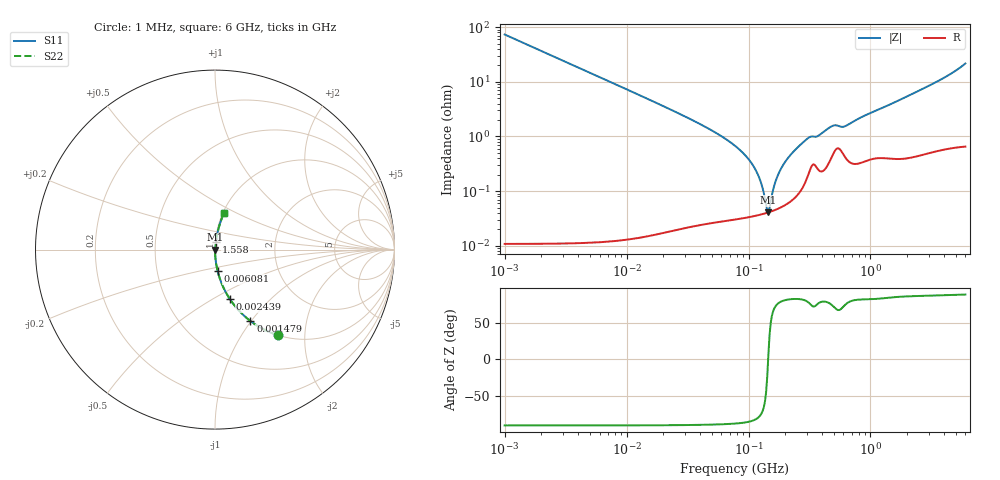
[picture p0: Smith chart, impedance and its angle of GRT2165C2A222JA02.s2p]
!Murata Part Number: GRT2165C2A222JA02
!These Parameters are Measured in Series Mode Connection
!Data Generated on Jun 19, 2026
!  o--ll--o
!Port1  Port2
!  o------o
!Operation Temp=25[degC], DC Bias Voltage=0[V]
!Freq. Start=1000[kHz] Stop=6[GHz] 401[Steps]
# Hz S RI R 50
!Freq.(Hz) S11(Real) S11(Imag) S21(Real) S21(Imag) S12(Real) S12(Imag) S22(Real) S22(Imag)
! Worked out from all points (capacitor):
!   401 points, 1 MHz to 6 GHz, reference 50 ohm
!   read as one part in series: C = 2.17 nF near 1.044 MHz
!   lowest |Z| = 41.2 mohm at 145.5 MHz (marker M1)
!   series resonance near 144.9 MHz, so ESL is about 560 pH
!   S11 on the Smith chart (normalised r, x): 1 MHz: 1.00, -1.47; 1.479 MHz: 1.00, -0.99; 2.439 MHz: 1.00, -0.60; 6.081 MHz: 1.00, -0.24; 1.558 GHz: 1.01, +0.08; 6 GHz: 1.01, +0.43
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1000000  0.35 -0.4769  0.65 0.4769  0.65 0.4769  0.35 -0.4769
1479166  0.1975 -0.398  0.8025 0.398  0.8025 0.398  0.1975 -0.398
2439274  0.083 -0.2758  0.917 0.2758  0.917 0.2758  0.083 -0.2758
4293785  0.0284 -0.1659  0.9716 0.1659  0.9716 0.1659  0.0284 -0.1659
6080879  0.0144 -0.1187  0.9856 0.1187  0.9856 0.1187  0.0144 -0.1187
1.843659e7  0.00169 -0.039  0.9983 0.039  0.9983 0.039  0.00169 -0.039
4.596069e7  0.000457 -0.0143  0.9995 0.0143  0.9995 0.0143  0.000457 -0.0143
7.745967e7  0.000348 -0.00674  0.9997 0.00674  0.9997 0.00674  0.000348 -0.00674
9.83954e7  0.000347 -0.00401  0.9997 0.00401  0.9997 0.00401  0.000347 -0.00401
1.145757e8  0.00036 -0.0024  0.9996 0.0024  0.9996 0.0024  0.00036 -0.0024
1.277378e8  0.000378 -0.00128  0.9996 0.00128  0.9996 0.00128  0.000378 -0.00128
1.39348e8  0.000397 -0.000394  0.9996 0.000394  0.9996 0.000394  0.000397 -0.000394
1.455431e8  0.000409 4.89e-05  0.9996 -4.89e-05  0.9996 -4.89e-05  0.000409 4.89e-05
1.694764e8  0.000466 0.00162  0.9995 -0.00162  0.9995 -0.00162  0.000466 0.00162
1.930997e8  0.000542 0.00301  0.9995 -0.00301  0.9995 -0.00301  0.000542 0.00301
2.506837e8  0.000874 0.00613  0.9991 -0.00613  0.9991 -0.00613  0.000874 0.00613
3.325952e8  0.00306 0.00951  0.9969 -0.00951  0.9969 -0.00951  0.00306 0.00951
4.919634e8  0.00487 0.0149  0.9951 -0.0149  0.9951 -0.0149  0.00487 0.0149
6.249308e8  0.00427 0.0149  0.9957 -0.0149  0.9957 -0.0149  0.00427 0.0149
1.428092e9  0.00533 0.0375  0.9947 -0.0375  0.9947 -0.0375  0.00533 0.0375
1.557894e9  0.00556 0.041  0.9944 -0.041  0.9944 -0.041  0.00556 0.041
6e9  0.0503 0.2041  0.9497 -0.2041  0.9497 -0.2041  0.0503 0.2041
